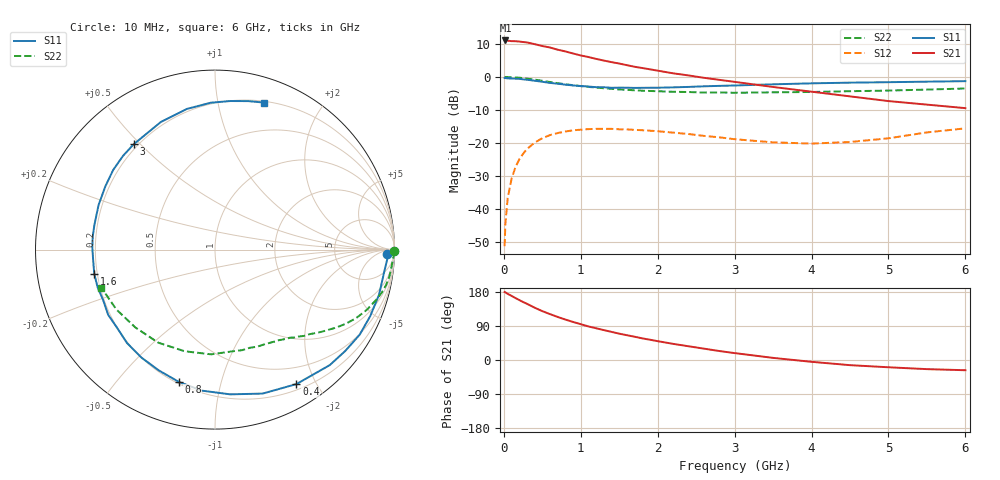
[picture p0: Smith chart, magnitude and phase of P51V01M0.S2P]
! SIEMENS Small Signal Semiconductors
! BFP183
! Si NPN RF Bipolar Junction Transistor in SOT143
! VCE = 1 V  IC = 1 mA
! Common Emitter S-Parameters:  March  1996
# GHz  S  MA  R  50
!  f  S11  S21  S12  S22
! GHz  MAG  ANG  MAG  ANG  MAG  ANG  MAG  ANG
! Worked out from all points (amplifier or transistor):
!   36 points, 10 MHz to 6 GHz, reference 50 ohm
!   highest |S21| = 11.1 dB at 20 MHz (marker M1)
!   |S21| within 3 dB of that: start of sweep to 737 MHz
!   unconditionally stable (mu >= 1): 2.417 GHz to end of sweep
!   at 250 MHz: K = 0.11, MSG = 17.0 dB, |S12| = -23.3 dB
!   at 1.4 GHz: K = 0.57, MSG = 10.1 dB, |S12| = -15.8 dB
!   at 6 GHz: K = 1.20, MAG = 0.4 dB, |S12| = -15.6 dB
!   S11 on the Smith chart (normalised r, x): 10 MHz: 35, -23; 400 MHz: 0.27, -1.74; 800 MHz: 0.21, -0.74; 1.6 GHz: 0.19, -0.10; 3 GHz: 0.18, +0.48; 6 GHz: 0.21, +1.36
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0.01  0.9614 -1.5  3.542 179.3  0.0027 86.8  0.9993 -0.6
0.02  0.961 -3.2  3.578 178.5  0.0059 86.3  0.9982 -1.2
0.05  0.9506 -7.7  3.549 174.6  0.0145 87.1  0.994 -2.9
0.1  0.9479 -15.4  3.493 169.2  0.0283 80.8  0.9872 -5.9
0.15  0.9409 -23.2  3.486 163.6  0.0425 75.6  0.9826 -8.9
0.25  0.9195 -37.9  3.388 153.0  0.0682 66.8  0.9599 -14.4
0.3  0.9072 -45.2  3.342 148.4  0.0803 62.7  0.9429 -17.0
0.4  0.8759 -58.8  3.147 138.1  0.1005 54.8  0.9104 -21.6
0.5  0.845 -71.7  2.945 129.0  0.1176 47.6  0.8743 -25.9
0.6  0.8109 -84.0  2.797 121.1  0.131 40.9  0.838 -29.5
0.8  0.7637 -105.4  2.439 106.7  0.1484 29.6  0.7738 -35.3
0.9  0.7424 -114.9  2.268 100.4  0.1547 24.9  0.7492 -37.7
1.1  0.7151 -133.3  2.004 88.6  0.1614 17.0  0.7052 -42.0
1.3  0.6974 -148.7  1.772 78.9  0.1629 9.9  0.673 -46.0
1.6  0.6862 -168.6  1.509 65.4  0.1599 2.0  0.6374 -51.1
1.9  0.685 173.8  1.305 53.5  0.1527 -4.3  0.6121 -56.7
2.2  0.6946 159.1  1.135 42.6  0.1428 -8.5  0.5955 -62.3
3  0.7414 127.7  0.842 18.2  0.1135 -11.7  0.5751 -79.9
3.5  0.7724 113.0  0.704 5.6  0.1017 -6.8  0.584 -92.1
4.5  0.8189 91.6  0.507 -13.6  0.1029 10.9  0.6073 -121.4
5.5  0.8477 77.4  0.38 -24.1  0.144 19.3  0.643 -148.8
6  0.8629 71.7  0.336 -27.0  0.1658 17.1  0.6676 -161.5
